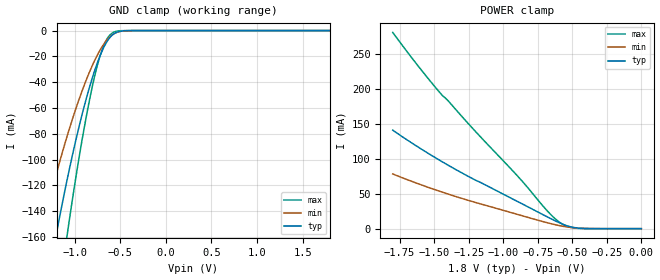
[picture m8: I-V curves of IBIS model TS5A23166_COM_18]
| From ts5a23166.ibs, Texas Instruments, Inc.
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[Model]   TS5A23166_COM_18
Model_type  Terminator
| variable   typ   min   max
C_comp   18.30pF   17.30pF   19.25pF
| C_tri-state   18.30pF   17.30pF   19.25pF
[Temperature Range]   40   100   -40
| Ambient temperature   25   85   -40
[Voltage range]   1.8   1.65   1.95
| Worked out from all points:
|   GND clamp passes 1 mA (typ) near -0.53 V on its own axis
|   POWER clamp passes 1 mA (typ) near -0.46 V on its own axis
[GND Clamp]
| TS5A23166_COM_18
|   Voltage   I(typ)   I(min)   I(max)
-1.8V     -424mA     -300.6mA   -592.3mA
-1.365V   -222.3mA   -156.3mA   -312.3mA
-1.195V   -155.1mA   -109.3mA   -216mA
-1.075V   -112.7mA   -79.82mA   -154.5mA
-930mV    -67.99mA   -48.81mA   -88.98mA
-855mV    -48.06mA   -34.98mA   -59.83mA
-790mV    -32.86mA   -24.42mA   -37.89mA
-735mV    -21.79mA   -16.71mA   -22.71mA
-680mV    -12.8mA    -10.35mA   -11.35mA
-580mV    -3.015mA   -2.912mA   -1.529mA
-400mV    -39.35uA   -69.37uA   -3.868uA
1.8V      606.3pA    485.3nA    44.83pA
[POWER Clamp]
| TS5A23166_COM_18
|   Voltage   I(typ)   I(min)   I(max)
-1.8V     140.9mA    78.21mA    280.7mA
-1.62V    117.2mA    64.55mA    233.7mA
-1.45V    96.63mA    52.78mA    192.6mA
-1.4V     90.89mA    49.53mA    183.2mA
-1.235V   72.9mA     39.43mA    146.4mA
-895mV    38.73mA    20.3mA     75.03mA
-680mV    16.8mA     8.401mA    25.23mA
-605mV    9.518mA    4.855mA    11.07mA
-545mV    4.603mA    2.664mA    3.913mA
-475mV    1.283mA    1.043mA    671.7uA
-370mV    98.84uA    142.3uA    21.44uA
-16.28fV  606.3pA    5.489nA    57.5pA
